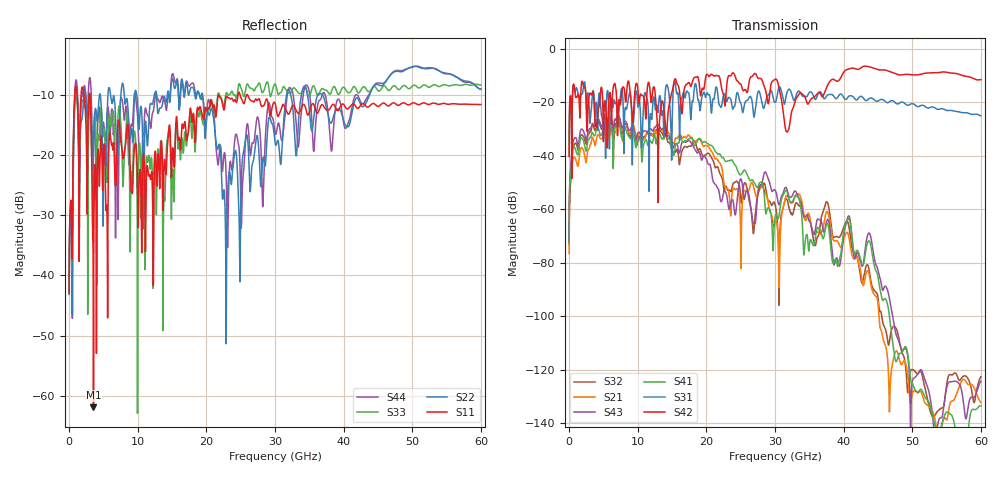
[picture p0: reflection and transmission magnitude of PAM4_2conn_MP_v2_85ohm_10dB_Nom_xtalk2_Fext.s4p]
! Info: Touchstone file created by Circ.  Input file=FAB50GbE_2conn_Midplane_Examax_Topo2_v2_85ohm_10dB_Nom.circ
# Hz S RI R 50
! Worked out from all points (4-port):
!   6000 points, 10 MHz to 60 GHz, reference 50 ohm
!   strongest paths, dB at 10 MHz, 15.01 GHz, 30.01 GHz, 45.01 GHz, 60 GHz:
!     S42: -40.2, -15.9, -11.3, -7.7, -11.4
!     S31: -39.9, -29.1, -19.9, -19.5, -25.0
!     S41: -72.8, -37.5, -62.9, -85.3, -133.6
!     S43: -71.6, -35.2, -52.8, -82.7, -124.4
!     S21: -76.6, -34.4, -65.2, -95.2, -132.3
!     S32: -73.4, -37.8, -58.1, -93.0, -122.7
!   lowest |S11| = -61.9 dB at 3.56 GHz (marker M1), VSWR 1.00, Z = 49.9 - j0.0459 ohm
!   |S11| at or under -10 dB: 3.041 GHz to 24.63 GHz (21.59 GHz wide, 156 % of centre); 24.91 GHz to 25.88 GHz (965.3 MHz wide, 3.8 % of centre); 25.99 GHz to end of sweep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
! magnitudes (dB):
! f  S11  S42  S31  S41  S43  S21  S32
! 10 MHz  -42.8  -40.2  -39.9  -72.8  -71.6  -76.6  -73.4
! 990 MHz  -8.6  -18.2  -14.8  -38.1  -33.2  -41.4  -35.2
! 3.56 GHz  -61.9  -16.8  -15.8  -32.2  -28.2  -33.8  -28.9
! 19.97 GHz  -12.2  -9.9  -17.6  -35.0  -41.0  -36.1  -39.5
! 31.78 GHz  -13.0  -31.0  -16.1  -53.6  -52.8  -54.8  -56.5
! 38.71 GHz  -11.9  -11.6  -18.2  -79.0  -80.1  -71.9  -70.5
! 60 GHz  -11.6  -11.4  -25.0  -133.6  -124.4  -132.3  -122.7
